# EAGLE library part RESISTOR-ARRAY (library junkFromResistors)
Array Chip Resistor Source: RS Component / Phycomp
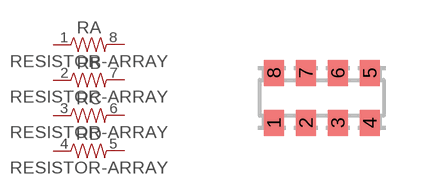
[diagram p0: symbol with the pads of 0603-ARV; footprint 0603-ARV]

Designator prefix R; gates A=RESISTOR-PADS B=RESISTOR-PADS C=RESISTOR-PADS D=RESISTOR-PADS

## RESISTOR-ARRAY0603-ARV  [0603-ARV]
1  A:1  pas
2  B:1  pas
3  C:1  pas
4  D:1  pas
5  D:2  pas
6  C:2  pas
7  B:2  pas
8  A:2  pas

## Footprint 0603-ARV (pad centres in mm)
Chip Resistor Array size 4 × 0603 convex termination - Phycomp Components Source: RS Components
smd 0.5 x 0.65: 1 -1.2,-0.625; 2 -0.4,-0.625; 3 0.4,-0.625; 4 1.2,-0.625; 5 1.2,0.625; 6 0.4,0.625; 7 -0.4,0.625; 8 -1.2,0.625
